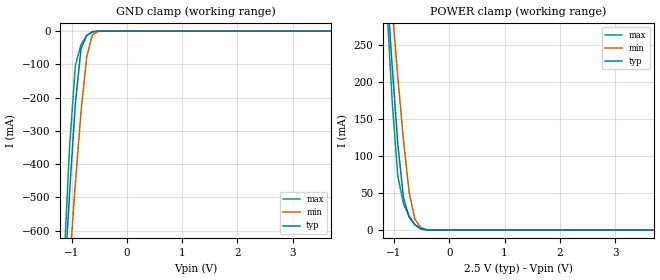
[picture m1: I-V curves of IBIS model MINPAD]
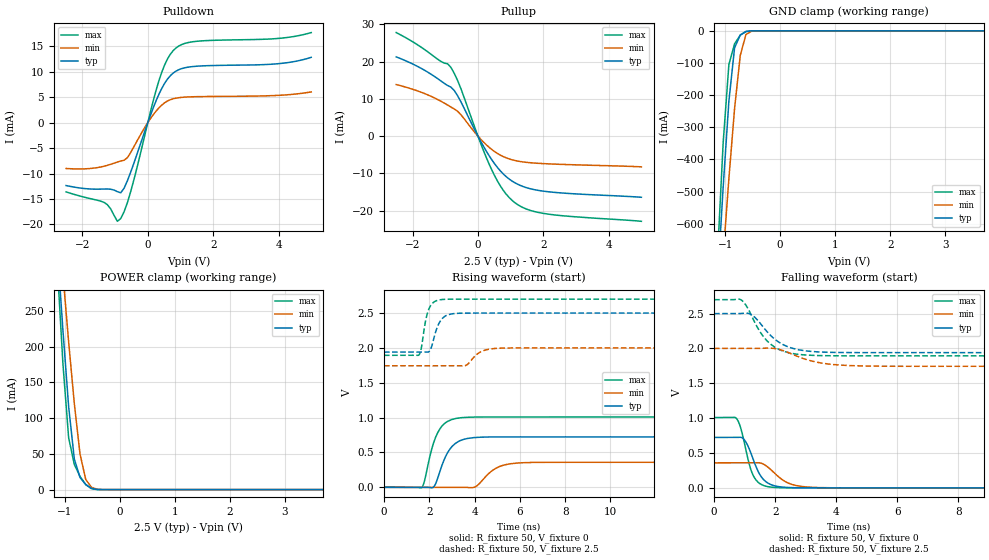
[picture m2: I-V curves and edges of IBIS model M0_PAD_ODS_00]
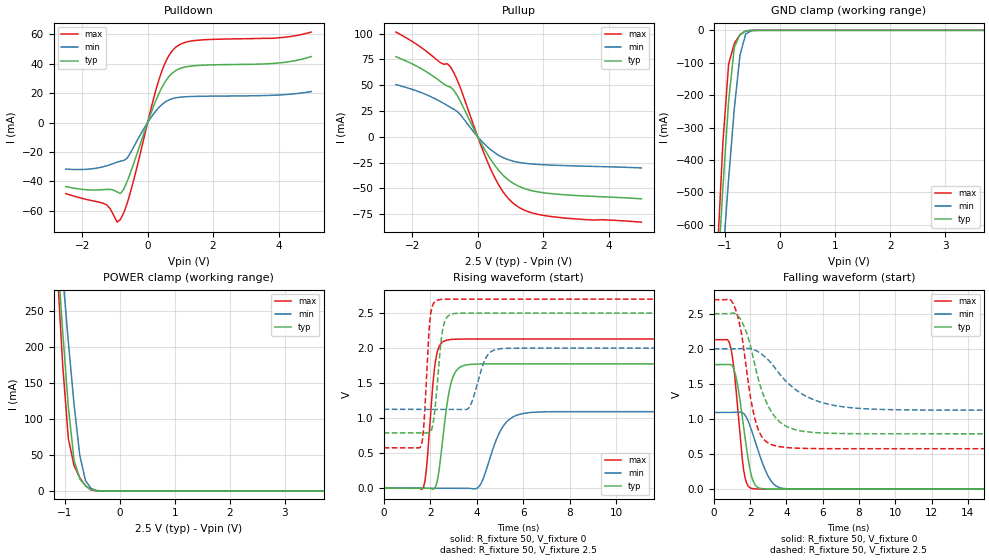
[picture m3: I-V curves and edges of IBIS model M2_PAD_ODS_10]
| Created by SiliconSmart  O-2018.09-SP2-3
[IBIS Ver]   4.0
[File Name]   as34b32bc_2p5_rev1p4.ibs
[File Rev]   1.4
[Date]   Thursday Mar 21 2024
|[Source]   Avalanche Team
|[Notes]   Generated IBIS models from Silicon Smart
|[Rev 1.0]  Initial Release based on extracted netlist
|   Characterization
|[Rev 1.1]  Recharacterization with Hspice, run in high accuracy mode
|[Rev 1.2]  Recharacterization with Hspice, parameters aligned with
|   datasheet
|[Rev 1.3]  Recharacterization with Hspice, run with updated VIH/VIL
|   in parallel with datasheet rev X.7
|[Rev 1.4]  Update the pin to the package pinout assignment
|[Disclaimer]   THE MODEL LIBRARIES ARE PROVIDED AS IS.
|[Copyright]   Copyright 2019, Avalanche Technology., All Rights Reserved
[Component]   AS304GB32_BGA
[Manufacturer] Avalanche Technology
| CONTENT :
| This file contains IBIS MODEL for PSRAM device
| AS304GB32
| USAGE :
| The models are derived for the 2.0V to 2.7V I/O Operation.
| Temperatures for model generation: typ: 25, max: -40, min: 125
| Voltages : typ: 2.5V, min: 2.0V, max: 2.7V
| PACKAGES SUPPORTED :
| 142-ball FBGA (15mm x 17mm)
| VERIFICATION
| Errors  : 0
| Warnings: 11
| All warnings due to non-monotonic data:
[Package]
R_pkg   0   0   0
L_pkg   0   0   0
C_pkg   0   0   0
[Pin]   signal_name   model_name   R_pin   L_pin   C_pin
P8   E#   MINPAD   0.254	7.307E-9	1.178E-12
P7   G#   MINPAD   0.243	7.052E-9	1.094E-12
J2   CR#   MINPAD   0.547	10.386E-9	1.789E-12
K3   PG#   MINPAD   0.451	10.329E-9	1.676E-12
M8   W#   MINPAD   0.377	9.020E-9	1.417E-12
M2   ADDR_26   MINPAD   0.425	9.037E-9	1.604E-12
L4   ADDR_25   MINPAD   0.419	9.644E-9	1.527E-12
K13   ADDR_24   MINPAD   0.495	9.978E-9	1.745E-12
M3   ADDR_23   MINPAD   0.371	9.313E-9	1.466E-12
L3   ADDR_22   MINPAD   0.412	9.753E-9	1.540E-12
M7   ADDR_21   MINPAD   0.368	8.765E-9	1.384E-12
P12   ADDR_20   MINPAD   0.287	8.287E-9	1.639E-12
L12   ADDR_19   MINPAD   0.424	10.320E-9	1.620E-12
N11   ADDR_18   MINPAD   0.338	8.691E-9	1.470E-12
N6   ADDR_17   MINPAD   0.309	8.196E-9	1.279E-12
P6   ADDR_16   MINPAD   0.256	7.462E-9	1.204E-12
L13   ADDR_15   MINPAD   0.463	10.719E-9	1.740E-12
M13   ADDR_14   MINPAD   0.421	10.290E-9	1.689E-12
P10   ADDR_13   MINPAD   0.262	7.671E-9	1.349E-12
N10   ADDR_12   MINPAD   0.340	8.540E-9	1.360E-12
M12   ADDR_11   MINPAD   0.402	9.876E-9	1.604E-12
N13   ADDR_10   MINPAD   0.399	9.819E-9	1.696E-12
L11   ADDR_9   MINPAD   0.443	9.732E-9	1.569E-12
M11   ADDR_8   MINPAD   0.436	9.682E-9	1.671E-12
P5   ADDR_7   MINPAD   0.253	7.464E-9	1.277E-12
P3   ADDR_6   MINPAD   0.279	8.031E-9	1.557E-12
N5   ADDR_5   MINPAD   0.313	8.320E-9	1.359E-12
N4   ADDR_4   MINPAD   0.329	8.138E-9	1.428E-12
M4   ADDR_3   MINPAD   0.379	8.543E-9	1.406E-12
N2   ADDR_2   MINPAD   0.378	9.572E-9	1.637E-12
N9   ADDR_1   MINPAD   0.315	8.416E-9	1.305E-12
M9   ADDR_0   MINPAD   0.403	9.225E-9	1.473E-12
E2   DQ_31   MIOPAD   0.365	8.798E-9	1.454E-12
F2   DQ_30   MIOPAD   0.418	9.057E-9	1.576E-12
D2   DQ_29   MIOPAD   0.358	8.697E-9	1.520E-12
E3   DQ_28   MIOPAD   0.348	8.812E-9	1.441E-12
E12   DQ_27   MIOPAD   0.327	8.506E-9	1.443E-12
D10   DQ_26   MIOPAD   0.309	7.715E-9	1.264E-12
C9   DQ_25   MIOPAD   0.279	7.395E-9	1.219E-12
C7   DQ_24   MIOPAD   0.252	6.802E-9	1.108E-12
G4   DQ_23   MIOPAD   0.455	10.071E-9	1.775E-12
G3   DQ_22   MIOPAD   0.457	10.100E-9	1.750E-12
F13   DQ_21   MIOPAD   0.377	9.387E-9	1.566E-12
D13   DQ_20   MIOPAD   0.295	8.231E-9	1.460E-12
C10   DQ_19   MIOPAD   0.293	7.553E-9	1.298E-12
E8   DQ_18   MIOPAD   0.393	8.323E-9	1.436E-12
F6   DQ_17   MIOPAD   0.425	8.913E-9	1.517E-12
E5   DQ_16   MIOPAD   0.379	8.982E-9	1.460E-12
E13   DQ_15   MIOPAD   0.363	8.555E-9	1.474E-12
G11   DQ_14   MIOPAD   0.475	9.536E-9	1.630E-12
E10   DQ_13   MIOPAD   0.404	8.563E-9	1.453E-12
F9   DQ_12   MIOPAD   0.409	9.347E-9	1.513E-12
C8   DQ_11   MIOPAD   0.257	6.782E-9	1.111E-12
C6   DQ_10   MIOPAD   0.238	7.000E-9	1.114E-12
D6   DQ_9   MIOPAD   0.292	7.776E-9	1.248E-12
D4   DQ_8   MIOPAD   0.305	7.782E-9	1.343E-12
G12   DQ_7   MIOPAD   0.502	10.055E-9	1.687E-12
C12   DQ_6   MIOPAD   0.275	7.857E-9	1.346E-12
D11   DQ_5   MIOPAD   0.286	7.835E-9	1.360E-12
D9   DQ_4   MIOPAD   0.306	8.035E-9	1.299E-12
E7   DQ_3   MIOPAD   0.384	8.178E-9	1.375E-12
C5   DQ_2   MIOPAD   0.231	6.786E-9	1.150E-12
D5   DQ_1   MIOPAD   0.307	7.698E-9	1.346E-12
C3   DQ_0   MIOPAD   0.267	7.420E-9	1.241E-12
G13   INT#   MIOPAD   0.480	10.704E-9	1.759E-12
F10   VSSIO   GND   NA   NA   NA
L10   VSSIO   GND   NA   NA   NA
E9   VSSIO   GND   NA   NA   NA
L9   VSSIO   GND   NA   NA   NA
F8   VSSIO   GND   NA   NA   NA
L8   VSSIO   GND   NA   NA   NA
F7   VSSIO   GND   NA   NA   NA
L7   VSSIO   GND   NA   NA   NA
E6   VSSIO   GND   NA   NA   NA
L6   VSSIO   GND   NA   NA   NA
G5   VSSIO   GND   NA   NA   NA
A14   VSS   GND   NA   NA   NA
B14   VSS   GND   NA   NA   NA
C14   VSS   GND   NA   NA   NA
H13   VSS   GND   NA   NA   NA
R14   VSS   GND   NA   NA   NA
T14   VSS   GND   NA   NA   NA
A13   VSS   GND   NA   NA   NA
T13   VSS   GND   NA   NA   NA
A12   VSS   GND   NA   NA   NA
G10   VSS   GND   NA   NA   NA
H10   VSS   GND   NA   NA   NA
J10   VSS   GND   NA   NA   NA
K10   VSS   GND   NA   NA   NA
F5   VSS   GND   NA   NA   NA
L5   VSS   GND   NA   NA   NA
A2   VSS   GND   NA   NA   NA
T2   VSS   GND   NA   NA   NA
A1   VSS   GND   NA   NA   NA
B1   VSS   GND   NA   NA   NA
R1   VSS   GND   NA   NA   NA
T1   VSS   GND   NA   NA   NA
F12   VCCIO   POWER   NA   NA   NA
J12   VCCIO   POWER   NA   NA   NA
E11   VCCIO   POWER   NA   NA   NA
M10   VCCIO   POWER   NA   NA   NA
D8   VCCIO   POWER   NA   NA   NA
N8   VCCIO   POWER   NA   NA   NA
D7   VCCIO   POWER   NA   NA   NA
N7   VCCIO   POWER   NA   NA   NA
M5   VCCIO   POWER   NA   NA   NA
E4   VCCIO   POWER   NA   NA   NA
F3   VCCIO   POWER   NA   NA   NA
J3   VCCIO   POWER   NA   NA   NA
C13   VCC   POWER   NA   NA   NA
P13   VCC   POWER   NA   NA   NA
D12   VCC   POWER   NA   NA   NA
N12   VCC   POWER   NA   NA   NA
C11   VCC   POWER   NA   NA   NA
F11   VCC   POWER   NA   NA   NA
H11   VCC   POWER   NA   NA   NA
J11   VCC   POWER   NA   NA   NA
K11   VCC   POWER   NA   NA   NA
P11   VCC   POWER   NA   NA   NA
C4   VCC   POWER   NA   NA   NA
F4   VCC   POWER   NA   NA   NA
H4   VCC   POWER   NA   NA   NA
J4   VCC   POWER   NA   NA   NA
K4   VCC   POWER   NA   NA   NA
P4   VCC   POWER   NA   NA   NA
D3   VCC   POWER   NA   NA   NA
N3   VCC   POWER   NA   NA   NA
C2   VCC   POWER   NA   NA   NA
P2   VCC   POWER   NA   NA   NA
| IOPAD
[Model Selector] MIOPAD
| Model Description
M0_PAD_ODS_00   ODS_00
M1_PAD_ODS_01   ODS_01
M2_PAD_ODS_10   ODS_10
M3_PAD_ODS_11   ODS_11
| Models and submodels in the file (5): MINPAD (Input), M0_PAD_ODS_00 (I/O), M2_PAD_ODS_10 (I/O), M1_PAD_ODS_01 (I/O), M3_PAD_ODS_11 (I/O)
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| INPAD
[Model] MINPAD
Model_type Input
Enable   Active-High
Vinl  =  0.7
Vinh  =  1.8
| Capacitance   typ   min   max
C_comp   6.242700e-12  5.875656e-12  6.826272e-12
| Variables   typ   min   max
[GND Clamp Reference]   0   0   0
[POWER Clamp Reference]   2.5   2   2.7
[Pulldown Reference]   0   0   0
[Pullup Reference]   2.5   2   2.7
[Temperature Range]   25   125   -40
[Voltage Range]   2.5   2   2.7
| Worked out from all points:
|   GND clamp passes 1 mA (typ) near -0.56 V on its own axis
|   POWER clamp passes 1 mA (typ) near -0.46 V on its own axis
[GND Clamp]
| Voltage   I(typ)   I(min)   I(max)
-2.5V     -5.188A    -4.586A    -6.153A
-1.138V   -783.9mA   -953.3mA   -701.6mA
-1.034V   -484.9mA   -700.5mA   -347mA
-931mV    -219.3mA   -459.7mA   -104.8mA
-827.6mV  -52.73mA   -241.7mA   -40.46mA
-724.1mV  -12.9mA    -76.61mA   -13.47mA
-620.7mV  -2.491mA   -11.2mA    -1.731mA
-517.2mV  -140.4uA   -1.281mA   -29.07uA
-413.8mV  -3.361uA   -98.11uA   -229.1nA
5V        0A         0A         0A
[POWER Clamp]
| Voltage   I(typ)   I(min)   I(max)
-2.5V     2.044A     1.82A      2.427A
-1.138V   339mA      399.6mA    314.6mA
-1.034V   222.7mA    301.1mA    175.8mA
-931mV    116.3mA    206.8mA    72.64mA
-827.6mV  42.71mA    120.3mA    35.15mA
-724.1mV  16.95mA    49.78mA    18.47mA
-620.7mV  7.083mA    14.35mA    7.103mA
-517.2mV  1.86mA     3.351mA    1.319mA
-413.8mV  190.6uA    480.6uA    44.77uA
-310.3mV  6.062uA    46.87uA    467.4nA
5V        0A         0A         0A
[Model] M0_PAD_ODS_00
Model_type I/O
Enable   Active-High
Vinl  =  0.7
Vinh  =  1.8
Vmeas =  1.25
Cref  =  30e-12
| Capacitance   typ   min   max
C_comp   6.259786e-12  5.891456e-12  6.837814e-12
| Variables   typ   min   max
[GND Clamp Reference]   0   0   0
[POWER Clamp Reference]   2.5   2   2.7
[Pulldown Reference]   0   0   0
[Pullup Reference]   2.5   2   2.7
[Temperature Range]   25   125   -40
[Voltage Range]   2.5   2   2.7
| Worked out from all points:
|   slope of the pulldown table from 0 to 0.375 V, typ, clamps not added: 62.2 ohm
|   slope of the pullup table from 0 to 0.375 V, typ, clamps not added: 65.8 ohm
|   GND clamp passes 1 mA (typ) near -0.56 V on its own axis
|   POWER clamp passes 1 mA (typ) near -0.46 V on its own axis
|   falling waveform, R_fixture 50, V_fixture 0: 20-80 % time 438ps typ, 623ps min, 353ps max; typ from 0.724 V to 0 V
|   falling waveform, R_fixture 50, V_fixture 2.5: 20-80 % time 815ps typ, 1.07ns min, 721ps max; typ from 2.5 V to 1.94 V
|   rising waveform, R_fixture 50, V_fixture 0: 20-80 % time 602ps typ, 765ps min, 549ps max; typ from 0 V to 0.724 V
|   rising waveform, R_fixture 50, V_fixture 2.5: 20-80 % time 358ps typ, 522ps min, 282ps max; typ from 1.94 V to 2.5 V
[GND Clamp]
| Voltage   I(typ)   I(min)   I(max)
-2.5V     -5.188A    -4.586A    -6.153A
-1.138V   -783.9mA   -953.3mA   -701.6mA
-1.034V   -484.9mA   -700.5mA   -347mA
-931mV    -219.3mA   -459.7mA   -104.8mA
-827.6mV  -52.73mA   -241.7mA   -40.47mA
-724.1mV  -12.9mA    -76.61mA   -13.47mA
-620.7mV  -2.491mA   -11.2mA    -1.732mA
-517.2mV  -140.5uA   -1.281mA   -29.11uA
-413.8mV  -3.362uA   -98.11uA   -229.5nA
5V        0A         0A         0A
[POWER Clamp]
| Voltage   I(typ)   I(min)   I(max)
-2.5V     2.044A     1.82A      2.427A
-1.138V   339mA      399.6mA    314.6mA
-1.034V   222.7mA    301.1mA    175.8mA
-931mV    116.3mA    206.8mA    72.64mA
-827.6mV  42.71mA    120.3mA    35.15mA
-724.1mV  16.95mA    49.78mA    18.47mA
-620.7mV  7.083mA    14.35mA    7.103mA
-517.2mV  1.86mA     3.351mA    1.319mA
-413.8mV  190.6uA    480.6uA    44.77uA
-310.3mV  6.062uA    46.87uA    467.4nA
5V        0A         0A         0A
[Pulldown]
| Voltage   I(typ)   I(min)   I(max)
-2.5V     -12.35mA   -9.004mA   -13.6mA
-1.345V   -13.04mA   -8.57mA    -15.65mA
-1.138V   -13.07mA   -8.191mA   -16.91mA
-931mV    -13.55mA   -7.74mA    -19.37mA
-827.6mV  -13.78mA   -7.539mA   -18.82mA
-517.2mV  -9.616mA   -5.796mA   -13.4mA
344.8mV   5.633mA    2.926mA    8.322mA
603.4mV   8.558mA    4.247mA    12.51mA
948.3mV   10.39mA    4.896mA    15.04mA
1.638V    11.13mA    5.111mA    16.04mA
3.99V     11.57mA    5.352mA    16.53mA
5V        12.82mA    6.029mA    17.68mA
[Pullup]
| Voltage   I(typ)   I(min)   I(max)
-2.5V     21.3mA     13.86mA    27.83mA
-1.552V   17.28mA    11.15mA    22.76mA
-827.6mV  13.17mA    7.825mA    18.5mA
-724.1mV  12.26mA    7.304mA    16.87mA
-517.2mV  9.175mA    5.726mA    12.68mA
86.21mV   -1.417mA   -831.8uA   -2.006mA
431mV     -6.444mA   -3.64mA    -9.217mA
775.9mV   -10.17mA   -5.503mA   -14.57mA
1.121V    -12.49mA   -6.527mA   -17.82mA
1.552V    -14.02mA   -7.108mA   -19.81mA
2.069V    -14.86mA   -7.416mA   -20.85mA
5V        -16.43mA   -8.255mA   -22.89mA
[Ramp]
dV/dt_r   0.434162/0.602046n  0.215384/0.765373n  0.605568/0.549215n
dV/dt_f   0.335982/0.815197n  0.153621/1.07305n  0.483841/0.721095n
R_load = 50
[Falling Waveform]
R_fixture = 50
V_fixture = 0
V_fixture_min = 0
V_fixture_max = 0
| Time   V(typ)   V(min)   V(max)
0s        723.6mV    359mV      1.009V
735ps     724.4mV    359.5mV    994.5mV
874.9ps   725.2mV    359.6mV    855.6mV
1.005ns   680.9mV    359.7mV    620.4mV
1.284ns   407mV      359.9mV    176.6mV
1.543ns   160.5mV    354mV      49.87mV
1.866ns   46.48mV    258.3mV    10.33mV
2.485ns   4.493mV    59.2mV     744.6uV
3.345ns   480.6uV    5.401mV    711.6uV
21.88ns   369.6nV    337.6nV    -77.16nV
[Falling Waveform]
R_fixture = 50
V_fixture = 2.5
V_fixture_min = 2
V_fixture_max = 2.7
| Time   V(typ)   V(min)   V(max)
0s        2.5V       2V         2.7V
877.9ps   2.502V     2.001V     2.699V
1.258ns   2.475V     2.001V     2.441V
1.581ns   2.323V     2.003V     2.191V
1.85ns    2.188V     2.004V     2.062V
2.368ns   2.033V     1.952V     1.948V
2.917ns   1.971V     1.857V     1.909V
3.74ns    1.945V     1.777V     1.896V
4.98ns    1.94V      1.748V     1.894V
21.88ns   1.94V      1.744V     1.894V
[Rising Waveform]
R_fixture = 50
V_fixture = 0
V_fixture_min = 0
V_fixture_max = 0
| Time   V(typ)   V(min)   V(max)
0s        10.92nV    333.3nV    10.24nV
1.672ns   -733.5uV   -456.6uV   -2.227mV
2.174ns   -673uV     -593.7uV   618.5mV
2.376ns   133.7mV    -648.8uV   785.4mV
2.807ns   495mV      -766.5uV   944.9mV
3.181ns   635.3mV    -868.8uV   988.3mV
4.008ns   714mV      3.518mV    1.008V
4.974ns   722.9mV    278.6mV    1.009V
5.954ns   723.2mV    349.9mV    1.009V
21.88ns   723.6mV    359mV      1.009V
[Rising Waveform]
R_fixture = 50
V_fixture = 2.5
V_fixture_min = 2
V_fixture_max = 2.7
| Time   V(typ)   V(min)   V(max)
0s        1.94V      1.744V     1.894V
1.548ns   1.941V     1.744V     1.901V
1.858ns   1.941V     1.744V     2.418V
1.999ns   1.949V     1.744V     2.57V
2.375ns   2.315V     1.744V     2.684V
2.593ns   2.428V     1.744V     2.695V
3.582ns   2.499V     1.745V     2.699V
4.251ns   2.5V       1.94V      2.699V
5.102ns   2.5V       1.996V     2.699V
21.88ns   2.5V       2V         2.7V
[Model] M2_PAD_ODS_10
Model_type I/O
Enable   Active-High
Vinl  =  0.7
Vinh  =  1.8
Vmeas =  1.25
Cref  =  30e-12
| Capacitance   typ   min   max
C_comp   6.259786e-12  5.891456e-12  6.837814e-12
| Variables   typ   min   max
[GND Clamp Reference]   0   0   0
[POWER Clamp Reference]   2.5   2   2.7
[Pulldown Reference]   0   0   0
[Pullup Reference]   2.5   2   2.7
[Temperature Range]   25   125   -40
[Voltage Range]   2.5   2   2.7
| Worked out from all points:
|   slope of the pulldown table from 0 to 0.375 V, typ, clamps not added: 17.8 ohm
|   slope of the pullup table from 0 to 0.375 V, typ, clamps not added: 18 ohm
|   GND clamp passes 1 mA (typ) near -0.56 V on its own axis
|   POWER clamp passes 1 mA (typ) near -0.46 V on its own axis
|   falling waveform, R_fixture 50, V_fixture 0: 20-80 % time 588ps typ, 895ps min, 457ps max; typ from 1.77 V to 0 V
|   falling waveform, R_fixture 50, V_fixture 2.5: 20-80 % time 1.21ns typ, 2.22ns min, 783ps max; typ from 2.5 V to 0.789 V
|   rising waveform, R_fixture 50, V_fixture 0: 20-80 % time 419ps typ, 751ps min, 304ps max; typ from 0 V to 1.77 V
|   rising waveform, R_fixture 50, V_fixture 2.5: 20-80 % time 280ps typ, 478ps min, 207ps max; typ from 0.789 V to 2.5 V
[GND Clamp]
| Voltage   I(typ)   I(min)   I(max)
-2.5V     -5.188A    -4.586A    -6.153A
-1.138V   -783.9mA   -953.3mA   -701.6mA
-1.034V   -484.9mA   -700.5mA   -347mA
-931mV    -219.3mA   -459.7mA   -104.8mA
-827.6mV  -52.73mA   -241.7mA   -40.47mA
-724.1mV  -12.9mA    -76.61mA   -13.47mA
-620.7mV  -2.491mA   -11.2mA    -1.732mA
-517.2mV  -140.5uA   -1.281mA   -29.11uA
-413.8mV  -3.362uA   -98.11uA   -229.5nA
5V        0A         0A         0A
[POWER Clamp]
| Voltage   I(typ)   I(min)   I(max)
-2.5V     2.044A     1.82A      2.427A
-1.138V   339mA      399.6mA    314.6mA
-1.034V   222.7mA    301.1mA    175.8mA
-931mV    116.3mA    206.8mA    72.64mA
-827.6mV  42.71mA    120.3mA    35.15mA
-724.1mV  16.95mA    49.78mA    18.47mA
-620.7mV  7.083mA    14.35mA    7.103mA
-517.2mV  1.86mA     3.351mA    1.319mA
-413.8mV  190.6uA    480.6uA    44.77uA
-310.3mV  6.062uA    46.87uA    467.4nA
5V        0A         0A         0A
[Pulldown]
| Voltage   I(typ)   I(min)   I(max)
-2.5V     -43.5mA    -31.6mA    -48.22mA
-1.345V   -45.55mA   -29.94mA   -54.89mA
-1.138V   -45.4mA    -28.55mA   -58.67mA
-931mV    -47.14mA   -26.9mA    -67.65mA
-827.6mV  -48.21mA   -26.21mA   -65.71mA
-517.2mV  -33.61mA   -20.26mA   -46.69mA
344.8mV   19.68mA    10.22mA    29mA
603.4mV   29.91mA    14.84mA    43.66mA
948.3mV   36.32mA    17.11mA    52.56mA
1.638V    38.89mA    17.86mA    56.1mA
3.99V     40.44mA    18.69mA    57.52mA
5V        44.82mA    21.06mA    61.44mA
[Pullup]
| Voltage   I(typ)   I(min)   I(max)
-2.5V     77.6mA     50.54mA    101.4mA
-1.552V   62.66mA    40.54mA    82.36mA
-1.138V   53.57mA    34.14mA    71.79mA
-827.6mV  48.05mA    28.38mA    67.64mA
-517.2mV  33.55mA    20.94mA    46.33mA
86.21mV   -5.181mA   -3.04mA    -7.328mA
431mV     -23.56mA   -13.31mA   -33.69mA
775.9mV   -37.17mA   -20.11mA   -53.29mA
1.121V    -45.67mA   -23.86mA   -65.22mA
1.552V    -51.29mA   -25.98mA   -72.55mA
2.155V    -54.68mA   -27.23mA   -76.79mA
5V        -59.99mA   -30.11mA   -82.63mA
[Ramp]
dV/dt_r   1.06496/0.418806n  0.655668/0.751369n  1.27778/0.303826n
dV/dt_f   1.02665/1.21101n  0.524479/2.21777n  1.27424/0.782834n
R_load = 50
[Falling Waveform]
R_fixture = 50
V_fixture = 0
V_fixture_min = 0
V_fixture_max = 0
| Time   V(typ)   V(min)   V(max)
0s        1.775V     1.093V     2.13V
740.7ps   1.776V     1.093V     2.131V
935.7ps   1.777V     1.093V     2.014V
1.234ns   1.588V     1.094V     1.394V
1.649ns   880.7mV    1.078V     267.9mV
2.029ns   241mV      878mV      15.26mV
2.371ns   33.92mV    605.8mV    2.475mV
3.019ns   1.942mV    172.9mV    492.1uV
3.736ns   490.1uV    14.78mV    372.9uV
21.88ns   -16.44nV   239.2nV    -101.2nV
[Falling Waveform]
R_fixture = 50
V_fixture = 2.5
V_fixture_min = 2
V_fixture_max = 2.7
| Time   V(typ)   V(min)   V(max)
0s        2.5V       2V         2.7V
856.7ps   2.501V     2V         2.708V
1.176ns   2.502V     2.001V     2.58V
1.482ns   2.417V     2.001V     2.279V
1.752ns   2.267V     2.007V     1.801V
2.269ns   1.762V     1.982V     999.3mV
3.127ns   1.123V     1.806V     640.9mV
4.9ns     825.6mV    1.351V     581.4mV
7.225ns   791.9mV    1.17V      576.5mV
21.88ns   788.9mV    1.126V     576.3mV
[Rising Waveform]
R_fixture = 50
V_fixture = 0
V_fixture_min = 0
V_fixture_max = 0
| Time   V(typ)   V(min)   V(max)
0s        5.137nV    182.5nV    4.377nV
1.709ns   -165.9uV   -473.8uV   13.88mV
1.851ns   -179.6uV   -513uV     321.1mV
2.22ns    14.43mV    -615.5uV   1.803V
2.685ns   1.113V     -744.3uV   2.112V
3.271ns   1.726V     -906.9uV   2.129V
4.101ns   1.773V     24.84mV    2.129V
5.037ns   1.774V     832.4mV    2.129V
6.039ns   1.774V     1.069V     2.129V
21.88ns   1.775V     1.093V     2.13V
[Rising Waveform]
R_fixture = 50
V_fixture = 2.5
V_fixture_min = 2
V_fixture_max = 2.7
| Time   V(typ)   V(min)   V(max)
0s        788.9mV    1.126V     576.3mV
1.615ns   788.4mV    1.126V     613.5mV
1.725ns   788.3mV    1.126V     894.7mV
1.998ns   795.3mV    1.126V     2.433V
2.34ns    1.636V     1.125V     2.689V
2.591ns   2.344V     1.125V     2.698V
2.997ns   2.491V     1.125V     2.7V
3.655ns   2.5V       1.144V     2.7V
4.923ns   2.5V       1.987V     2.7V
21.88ns   2.5V       2V         2.7V
